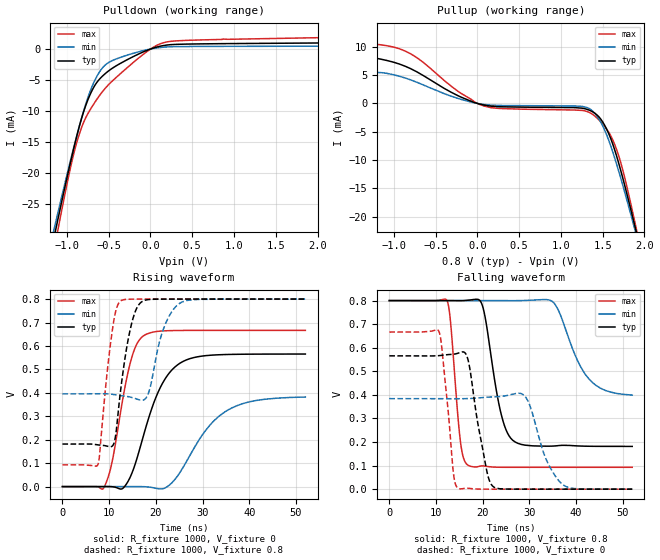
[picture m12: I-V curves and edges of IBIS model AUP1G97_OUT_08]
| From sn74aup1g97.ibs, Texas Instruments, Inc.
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[Model]   AUP1G97_OUT_08
Model_type  Output
Vref =   0
Rref =   1E6
Cref =   30p
Vmeas =   0.4
| variable   typ   min   max
C_comp   2.62pF   2.11pF   3.26pF
| C_pullup   2.68pF   2.11pF   3.26pF
| C_pulldown   2.55pF   2.11pF   2.99pF
[Temperature Range]   40   100   -40
| Ambient temperature   25   85   -40
[Voltage range]   0.8   0.8   0.8
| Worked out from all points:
|   slope of the pulldown table from 0 to 0.12 V, typ, clamps not added: 257 ohm
|   slope of the pullup table from 0 to 0.12 V, typ, clamps not added: 309 ohm
|   rising waveform, R_fixture 1000, V_fixture 0: 20-80 % time 5.92ns typ, 8.21ns min, 3.69ns max; typ from 0 V to 0.566 V
|   falling waveform, R_fixture 1000, V_fixture 0.8: 20-80 % time 3.16ns typ, 5.26ns min, 1.71ns max; typ from 0.8 V to 0.181 V
|   rising waveform, R_fixture 1000, V_fixture 0.8: 20-80 % time 2.71ns typ, 3.28ns min, 2.25ns max; typ from 0.181 V to 0.8 V
|   falling waveform, R_fixture 1000, V_fixture 0: 20-80 % time 2.83ns typ, 4.03ns min, 1.84ns max; typ from 0.566 V to 0 V
[Pulldown]
| AUP1G97_OUT_08
|   Voltage   I(typ)   I(min)   I(max)
-3.6V     -200.3mA   -184.7mA   -219.1mA
-1.155V   -30.43mA   -29.11mA   -32.45mA
-1.105V   -27.26mA   -26.22mA   -28.93mA
-940mV    -17.24mA   -17.01mA   -18.09mA
-865mV    -13.13mA   -13.1mA    -14.27mA
-745mV    -8.043mA   -7.657mA   -10.32mA
-630mV    -5.174mA   -4.128mA   -7.88mA
-470mV    -3.218mA   -1.946mA   -5.328mA
5mV       23.8uA     12.51uA    45.54uA
245mV     711.3uA    371.9uA    1.246mA
870mV     872.1uA    431.7uA    1.618mA
7.2V      1.459mA    578.6uA    3.138mA
[Pullup]
| AUP1G97_OUT_08
|   Voltage   I(typ)   I(min)   I(max)
-3.6V     2.784mA    339.2uA    9.474mA
-2.56V    3.921mA    663.8uA    11.14mA
-2.01V    6.261mA    1.269mA    13.37mA
-1.185V   7.906mA    5.477mA    10.41mA
-800mV    6.149mA    4.169mA    8.776mA
80mV      -287uA     -177.3uA   -461.9uA
1.285V    -921uA     -607uA     -1.305mA
1.455V    -2.355mA   -2.736mA   -2.902mA
1.625V    -7.333mA   -8.725mA   -6.56mA
1.74V     -13.09mA   -14.38mA   -11.68mA
1.905V    -22.78mA   -23.32mA   -22.23mA
7.2V      -396.8mA   -367.4mA   -431.7mA
[Ramp]
| AUP1G97_OUT_08
| variable   typ   min   max
dV/dt_r   0.35/5.99E-09   0.24/8.32E-09   0.41/3.74E-09
dV/dt_f   0.37/3.17E-09   0.24/5.28E-09   0.43/1.72E-09
R_load = 1000
[Rising Waveform]
| AUP1G97_OUT_08
R_fixture =   1000
C_fixture =   0
L_fixture =   0
V_fixture =   0
V_fixture_min = 0
V_fixture_max = 0
|   Time   V(typ)   V(min)   V(max)
0s        23.71nV    153.5nV    1.008nV
8.915ns   138.8uV    32.11uV    -2.8mV
10.65ns   -521.3uV   166.9uV    106.8mV
13.41ns   3.01mV     60.19uV    427.4mV
15.36ns   83.32mV    191.6uV    582.3mV
17.47ns   226.3mV    -394.7uV   644.7mV
21.38ns   439.1mV    -9.386mV   663.9mV
25.94ns   535.1mV    85.68mV    666.2mV
35.49ns   563.6mV    327.3mV    666.5mV
52ns      565.5mV    382.1mV    666.5mV
[Falling Waveform]
| AUP1G97_OUT_08
R_fixture =   1000
C_fixture =   0
L_fixture =   0
V_fixture =   0.8
V_fixture_min = 0.8
V_fixture_max = 0.8
|   Time   V(typ)   V(min)   V(max)
0s        800mV      800mV      800mV
12.37ns   799.9mV    800mV      799.4mV
15.24ns   799.6mV    800mV      200.9mV
16.81ns   801.4mV    800mV      102mV
19.94ns   778.1mV    799.9mV    98.69mV
23.71ns   338.2mV    799.9mV    92.95mV
26.41ns   207.7mV    799.7mV    92.74mV
34.94ns   182.7mV    795.4mV    92.72mV
42.63ns   182.1mV    470mV      92.72mV
52ns      181.5mV    399.1mV    92.72mV
[Rising Waveform]
| AUP1G97_OUT_08
R_fixture =   1000
C_fixture =   0
L_fixture =   0
V_fixture =   0.8
V_fixture_min = 0.8
V_fixture_max = 0.8
|   Time   V(typ)   V(min)   V(max)
0s        181.5mV    395.5mV    92.72mV
7.64ns    177.9mV    396.1mV    96.36mV
10.99ns   182.6mV    392.8mV    705.9mV
12.52ns   420.8mV    387.9mV    792.6mV
14.85ns   698.8mV    380.2mV    799.7mV
17.28ns   791.9mV    368.9mV    799.9mV
18.64ns   798.2mV    412.8mV    800mV
21.78ns   799.8mV    680.6mV    800mV
25.13ns   800mV      782.3mV    800mV
52ns      800mV      800mV      800mV
[Falling Waveform]
| AUP1G97_OUT_08
R_fixture =   1000
C_fixture =   0
L_fixture =   0
V_fixture =   0
V_fixture_min = 0
V_fixture_max = 0
|   Time   V(typ)   V(min)   V(max)
0s        565.5mV    384mV      666.5mV
10.63ns   566.4mV    383.8mV    668.7mV
13.74ns   572.5mV    383.6mV    66.23mV
14.71ns   576.8mV    383.6mV    4.249mV
16.83ns   550.4mV    384.3mV    3.905mV
20.77ns   87.16mV    389.8mV    50.23uV
22.27ns   10.32mV    391.5mV    8.513uV
29.11ns   24.08uV    392.3mV    -41.81nV
37.3ns    195nV      16.92mV    -102.2nV
52ns      -1.029uV   4.425uV    -460.1nV
